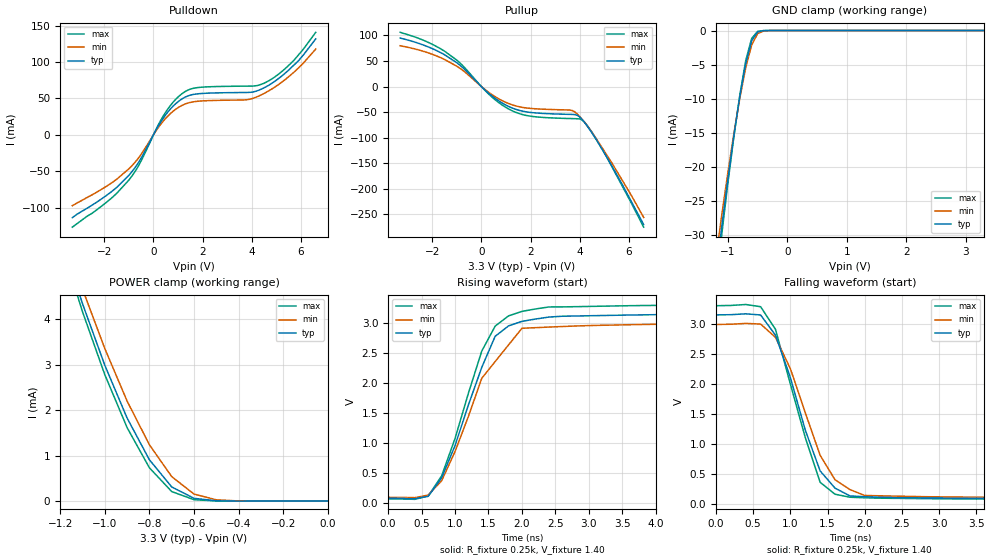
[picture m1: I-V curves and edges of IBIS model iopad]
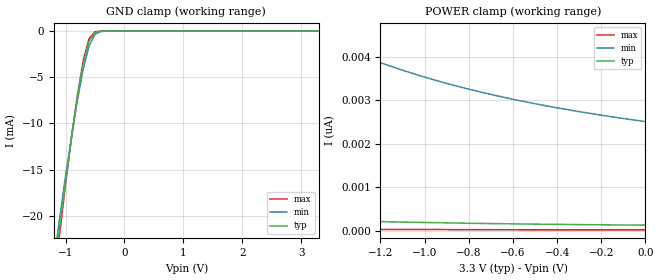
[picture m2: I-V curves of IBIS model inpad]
| IBIS file 70v3579.ibs created by s2ibis2 version 1.1
| North Carolina State University Electronics Research Laboratory  1995
[IBIS ver]   2.1
[File name]   70v3579.ibs
[File Rev]   1.0
[Date]   12/16/98 mff
[Source]   Integrated Device Technology, Inc.
[Notes]   1.Temperatures: typ=25C, min=70C, max=0C 2.RRmp rates based on
   50 ohm load.
[Disclaimer] Integrated Device Technology, Inc. ("IDT") hereby grants the
   user of this IBIS model a non-exclusive, nontransferable
   license to use this IBIS model under the following terms. The
   user is granted this license only to use the IBIS model and is
   not granted rights to sell, copy (except as needed to run the
   IBIS model), rent, lease or sub-license the IBIS model in
   whole or in part, or in modified form to anyone. The User may
   modify the IBIS model to suit its specific applications, but
   rights to derivative works and such modifications shall belong
   to IDT. This IBIS model is provided on an AS IS" basis and IDT
   makes absolutely no warranty with respect to the information
   contained herein. IDT DISCLAIMS AND CUSTOMER WAIVES ALL
   WARRANTIES, EXPRESS AND IMPLIED, INCLUDING WARRANTIES OF
   MERCHANTABILITY AND FITNESS FOR A PARTICULAR PURPOSE. THE
   ENTIRE RISK AS TO QUALITY AND PERFORMANCE IS WITH THE USER
   ACCORDINGLY, IN NO EVENT SHALL IDT BE LIABLE FOR ANY DIRECT OR
   INDIRECT DAMAGES, WHETHER IN CONTRACT OR TORT, INCLUDING ANY
   LOST PROFITS OR OTHER INCIDENTAL, CONSEQUENTIAL, EXEMPLARY, OR
   PUNITIVE DAMAGES ARISING OUT OF THE USE OR APPLICATION OF THE
   IBIS model. Further, IDT reserves the right to make changes
   without notice to any product herein to improve reliability,
   function, or design. IDT does not convey any license under
   patent rights or any other intellectual property rights,
   including those of third parties. IDT is not obligated to
   provide maintenance or support for the licensed IBIS model.
[Copyright]   Copyright 1998, Integrated Device Technology, Inc. all rights
   reserved
|   Component 70v3579dr208
[Component]   70v3579dr208
[Manufacturer]   Integrated Device Technology
[Package]
| variable   typ   min   max
R_pkg   100.00m   50.00m   0.30
L_pkg   12.00nH   10.00nH   14.00nH
C_pkg   2.80pF   1.50pF   6.00pF
[Pin]  signal_name   model_name   R_pin   L_pin   C_pin
1   io19l   iopad
2   io19r   iopad
3   io20l   iopad
4   io20r   iopad
5   vddql   POWER
6   vss   GND
7   io21l   iopad
8   io21r   iopad
9   io22l   iopad
10   io22r   iopad
11   vddqr   POWER
12   vss   GND
13   io23l   iopad
14   io23r   iopad
15   io24l   iopad
16   io24r   iopad
17   vddql   POWER
18   vss   GND
19   io25l   iopad
20   io25r   iopad
21   io26l   iopad
22   io26r   iopad
23   vddqr   POWER
24   vss   GND
25   vdd   POWER
26   vdd   POWER
27   vss   GND
28   vss   GND
29   vddql   POWER
30   vss   GND
31   io27r   iopad
32   io27l   iopad
33   io28r   iopad
34   io28l   iopad
35   vddqr   POWER
36   vss   GND
37   io29r   iopad
38   io29l   iopad
39   io30r   iopad
40   io30l   iopad
41   vddql   POWER
42   vss   GND
43   io31r   iopad
44   io31l   iopad
45   io32r   iopad
46   io32l   iopad
47   vddqr   POWER
48   vss   GND
49   io33r   iopad
50   io33l   iopad
51   io34r   iopad
52   io34l   iopad
53   vss   GND
54   vddql   POWER
55   io35r   iopad
56   io35l   iopad
57   vdd   POWER
58   vss   GND
66   a14r   inpad
67   a13r   inpad
68   a12r   inpad
69   a11r   inpad
70   a10r   inpad
71   a9r   inpad
72   a8r   inpad
73   a7r   inpad
74   be3r#   inpad
75   be2r#   inpad
76   be1r#   inpad
77   be0r#   inpad
78   ce1r   inpad
79   ce0r   inpad
80   vdd   POWER
81   vdd   POWER
82   vss   GND
83   vss   GND
84   clkr   inpad
85   oer#   inpad
86   rwr#   inpad
87   adsr#   inpad
88   cntenr#   inpad
89   cntrstr#   inpad
90   a6r   inpad
91   a5r   inpad
92   a4r   inpad
93   a3r   inpad
94   a2r   inpad
95   a1r   inpad
96   a0r   inpad
97   vdd   POWER
98   vss   GND
99   vss   GND
100   vdd   POWER
101   io0l   iopad
102   io0r   iopad
103   vddql   POWER
104   vss   GND
105   io1l   iopad
106   io1r   iopad
107   io2l   iopad
108   io2r   iopad
109   vddqr   POWER
110   vss   GND
111   io3l   iopad
112   io3r   iopad
113   io4l   iopad
114   io4r   iopad
115   vddql   POWER
116   vss   GND
117   io5l   iopad
118   io5r   iopad
119   io6l   iopad
120   io6r   iopad
121   vddqr   POWER
122   vss   GND
123   io7l   iopad
124   io7r   iopad
125   io8l   iopad
126   io8r   iopad
127   vddql   POWER
128   vss   GND
129   vss   GND
130   vss   GND
131   vdd   POWER
132   vdd   POWER
133   vddqr   POWER
134   vss   GND
135   io9r   iopad
136   io9l   iopad
137   io10r   iopad
138   io10l   iopad
139   vddql   POWER
140   vss   GND
141   io11r   iopad
142   io11l   iopad
143   io12r   iopad
144   io12l   iopad
145   vddqr   POWER
146   vss   GND
147   io13r   iopad
148   io13l   iopad
149   io14r   iopad
150   io14l   iopad
151   vddql   POWER
152   vss   GND
153   io15r   iopad
154   io15l   iopad
155   io16r   iopad
156   io16l   iopad
157   vss   GND
158   vddqr   POWER
159   io17r   iopad
160   io17l   iopad
161   vdd   POWER
162   vss   GND
163   vdd   POWER
164   vdd   POWER
165   a0l   inpad
166   a1l   inpad
167   a2l   inpad
168   a3l   inpad
169   a4l   inpad
170   a5l   inpad
171   a6l   inpad
172   cntrstl#   inpad
173   cntenl#   inpad
174   adsl#   inpad
175   rwl#   inpad
176   oel#   inpad
177   clkl   inpad
178   vss   GND
179   vss   GND
180   vdd   POWER
181   vdd   POWER
182   ce0l   inpad
183   ce1l   inpad
184   be0l#   inpad
185   be1l#   inpad
186   be2l#   inpad
187   be3l#   inpad
188   a7l   inpad
189   a8l   inpad
190   a9l   inpad
191   a10l   inpad
192   a11l   inpad
193   a12l   inpad
194   a13l   inpad
195   a14l   inpad
202   vss   GND
203   vdd   POWER
204   vss   GND
205   io18l   iopad
206   io18r   iopad
207   vddqr   POWER
208   vss   GND
| in   in   dummy_model
| oe   oe   dummy_model
[Pin Mapping]  pulldown_ref   pullup_ref   gnd_clamp_ref   power_clamp_ref
1   vss   vddql
2   vss   vddqr
3   vss   vddql
4   vss   vddqr
5   NC   vddql
6   vss   NC
7   vss   vddql
8   vss   vddqr
9   vss   vddql
10   vss   vddqr
11   NC   vddqr
12   vss   NC
13   vss   vddql
14   vss   vddqr
15   vss   vddql
16   vss   vddqr
17   NC   vddql
18   vss   NC
19   vss   vddql
20   vss   vddqr
21   vss   vddql
22   vss   vddqr
23   NC   vddqr
24   vss   NC
25   NC   vdd
26   NC   vdd
27   vss   NC
28   vss   NC
29   NC   vddql
30   vss   NC
31   vss   vddqr
32   vss   vddql
33   vss   vddqr
34   vss   vddql
35   NC   vddqr
36   vss   NC
37   vss   vddqr
38   vss   vddql
39   vss   vddqr
40   vss   vddql
41   NC   vddql
42   vss   NC
43   vss   vddqr
44   vss   vddql
45   vss   vddqr
46   vss   vddql
47   NC   vddqr
48   vss   NC
49   vss   vddqr
50   vss   vddql
51   vss   vddqr
52   vss   vddql
53   vss   NC
54   NC   vddql
55   vss   vddqr
56   vss   vddql
57   NC   vdd
58   vss   NC
66   vss   vdd
67   vss   vdd
68   vss   vdd
69   vss   vdd
70   vss   vdd
71   vss   vdd
72   vss   vdd
73   vss   vdd
74   vss   vdd
75   vss   vdd
76   vss   vdd
77   vss   vdd
78   vss   vdd
79   vss   vdd
80   NC   vdd
81   NC   vdd
82   vss   NC
83   vss   NC
84   vss   vdd
85   vss   vdd
86   vss   vdd
87   vss   vdd
88   vss   vdd
89   vss   vdd
90   vss   vdd
91   vss   vdd
92   vss   vdd
93   vss   vdd
94   vss   vdd
95   vss   vdd
96   vss   vdd
97   NC   vdd
98   vss   NC
99   vss   NC
100   NC   vdd
101   vss   vddql
102   vss   vddqr
103   NC   vddql
104   vss   NC
105   vss   vddql
106   vss   vddqr
107   vss   vddql
108   vss   vddqr
109   NC   vddqr
110   vss   NC
111   vss   vddql
112   vss   vddqr
113   vss   vddql
114   vss   vddqr
115   NC   vddql
116   vss   NC
117   vss   vddql
118   vss   vddqr
119   vss   vddql
120   vss   vddqr
121   NC   vddqr
122   vss   NC
123   vss   vddql
124   vss   vddqr
125   vss   vddql
126   vss   vddqr
127   NC   vddql
128   vss   NC
129   vss   NC
130   vss   NC
131   NC   vdd
132   NC   vdd
133   NC   vddqr
134   vss   NC
135   vss   vddqr
136   vss   vddql
137   vss   vddqr
138   vss   vddql
139   NC   vddql
140   vss   NC
141   vss   vddqr
142   vss   vddql
143   vss   vddqr
144   vss   vddql
145   NC   vddqr
146   vss   NC
147   vss   vddqr
148   vss   vddql
149   vss   vddqr
150   vss   vddql
151   NC   vddql
152   vss   NC
153   vss   vddqr
154   vss   vddql
155   vss   vddqr
156   vss   vddql
157   vss   NC
158   NC   vddqr
159   vss   vddqr
160   vss   vddql
161   NC   vdd
162   vss   NC
163   NC   vdd
164   NC   vdd
165   vss   vdd
166   vss   vdd
167   vss   vdd
168   vss   vdd
169   vss   vdd
170   vss   vdd
171   vss   vdd
172   vss   vdd
173   vss   vdd
174   vss   vdd
175   vss   vdd
176   vss   vdd
177   vss   vdd
178   vss   NC
179   vss   NC
180   NC   vdd
181   NC   vdd
182   vss   vdd
183   vss   vdd
184   vss   vdd
185   vss   vdd
186   vss   vdd
187   vss   vdd
188   vss   vdd
189   vss   vdd
190   vss   vdd
191   vss   vdd
192   vss   vdd
193   vss   vdd
194   vss   vdd
195   vss   vdd
202   vss   NC
203   NC   vdd
204   vss   NC
205   vss   vddql
206   vss   vddqr
207   NC   vddqr
208   vss   NC
| Models and submodels in the file (2): iopad (I/O), inpad (Input)
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|in   NC   NC
|oe   NC   NC
|   Model iopad
[Model]   iopad
Model_type   I/O
Polarity   Non-Inverting
Enable   Active-High
Vinl =  0.800V
Vinh =  2.000V
Vmeas =  1.500V
C_comp   1.00pF   NA   NA
[Temperature Range]   25.00   70.00   0.000
[Voltage Range]   3.30V   3.15V   3.45V
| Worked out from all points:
|   slope of the pulldown table from 0 to 0.495 V, typ, clamps not added: 18 ohm
|   slope of the pullup table from 0 to 0.495 V, typ, clamps not added: 23.7 ohm
|   GND clamp passes 1 mA (typ) near -0.56 V on its own axis
|   POWER clamp passes 1 mA (typ) near -0.81 V on its own axis
|   rising waveform, R_fixture 0.25k, V_fixture 1.40: 20-80 % time 605ps typ, 716ps min, 576ps max; typ from 0.082 V to 3.15 V
|   falling waveform, R_fixture 0.25k, V_fixture 1.40: 20-80 % time 479ps typ, 525ps min, 448ps max; typ from 3.15 V to 0.082 V
[Pulldown]
| voltage   I(typ)   I(min)   I(max)
-3.3V     -114mA     -97.5mA    -127mA
-1.9V     -83.06mA   -70.53mA   -92.53mA
-1V       -55.69mA   -46.78mA   -62.24mA
-600mV    -37.64mA   -31.5mA    -42.12mA
400mV     22.98mA    18.97mA    26.02mA
1.1V      48.05mA    39.4mA     54.97mA
1.8V      56.39mA    46.16mA    65mA
3.8V      58.27mA    48.27mA    67mA
4.5V      64.64mA    56.89mA    71.01mA
5.1V      77.7mA     69.5mA     83.74mA
5.7V      95.54mA    85.76mA    102mA
6.6V      132mA      118mA      141mA
[Pullup]
| voltage   I(typ)   I(min)   I(max)
-3.3V     94.72mA    79.74mA    106mA
-2.3V     80.13mA    68mA       89.32mA
-1.5V     62.22mA    52.99mA    69.19mA
-800mV    38.7mA     33.19mA    42.88mA
400mV     -17.28mA   -14.82mA   -19.29mA
1.2V      -40.94mA   -34.88mA   -46.19mA
2V        -50.67mA   -42.77mA   -58.01mA
3.6V      -54.45mA   -46.05mA   -62.6mA
4V        -59.66mA   -58.71mA   -63.48mA
4.3V      -76.87mA   -76.45mA   -75.79mA
4.9V      -122mA     -119mA     -121mA
6.6V      -270mA     -256mA     -275mA
[GND_clamp]
| voltage   I(typ)   I(min)   I(max)
-3.3V     -213mA     -195mA     -224mA
-1.2V     -35.67mA   -33.21mA   -37.24mA
-1.1V     -28.54mA   -26.85mA   -29.61mA
-1V       -21.76mA   -20.81mA   -22.35mA
-900mV    -15.43mA   -15.14mA   -15.59mA
-800mV    -9.676mA   -9.946mA   -9.478mA
-700mV    -4.805mA   -5.441mA   -4.393mA
-600mV    -1.485mA   -2.103mA   -1.146mA
-500mV    -215uA     -458uA     -124uA
-400mV    -17.97uA   -58.09uA   -7.861uA
-300mV    -1.106uA   -5.62uA    -349nA
3.3V      143pA      13.86nA    17.08pA
[POWER_clamp]
| voltage   I(typ)   I(min)   I(max)
-3.3V     54.48mA    50.56mA    57.22mA
-1.2V     5.852mA    6.099mA    5.729mA
-1.1V     4.338mA    4.66mA     4.161mA
-1V       2.985mA    3.352mA    2.778mA
-900mV    1.825mA    2.198mA    1.615mA
-800mV    908uA      1.238mA    732uA
-700mV    312uA      538uA      210uA
-600mV    61.42uA    155uA      31.29uA
-500mV    7.539uA    28.27uA    3.013uA
-400mV    726nA      3.93uA     220nA
0V        143pA      2.833nA    18.39pA
[Ramp]
| variable   typ   min   max
dV/dt_r   1.24/1.42n   1.10/1.61n   1.37/1.50n
dV/dt_f   1.37/1.27n   1.20/1.54n   1.50/1.16n
R_load = 50.00
[Rising Waveform]
R_fixture = 0.25k
V_fixture = 1.40
| time   V(typ)   V(min)   V(max)
0s        81.93mV    98.35mV    72.87mV
600ps     115mV      136mV      121mV
800ps     421mV      373mV      454mV
1ns       956mV      858mV      1.074V
1.4ns     2.258V     2.076V     2.528V
1.6ns     2.773V     2.353V     2.942V
1.8ns     2.946V     2.63V      3.112V
2ns       3.021V     2.906V     3.187V
2.4ns     3.092V     2.926V     3.26V
19.8ns    3.148V     2.988V     3.301V
[Falling Waveform]
R_fixture = 0.25k
V_fixture = 1.40
| time   V(typ)   V(min)   V(max)
0s        3.148V     2.988V     3.301V
600ps     3.146V     2.995V     3.284V
800ps     2.81V      2.773V     2.907V
1ns       2.103V     2.251V     1.994V
1.2ns     1.229V     1.519V     1.105V
1.4ns     547mV      807mV      358mV
1.6ns     260mV      400mV      158mV
1.8ns     130mV      236mV      108mV
3.8ns     87.38mV    105mV      76.98mV
19.8ns    81.93mV    98.32mV    72.85mV
|   Model inpad
[Model]   inpad
Model_type   Input
Vinl =  0.800V
Vinh =  2.000V
C_comp   1.00pF   NA   NA
[Temperature Range]   25.00   70.00   0.000
[Voltage Range]   3.30V   3.15V   3.45V
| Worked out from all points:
|   GND clamp passes 1 mA (typ) near -0.59 V on its own axis
[GND_clamp]
| voltage   I(typ)   I(min)   I(max)
-3.3V     -151mA     -139mA     -158mA
-1.2V     -26.48mA   -24.89mA   -27.46mA
-1.1V     -21.24mA   -20.19mA   -21.89mA
-1V       -16.24mA   -15.68mA   -16.56mA
-900mV    -11.52mA   -11.43mA   -11.55mA
-800mV    -7.21mA    -7.515mA   -6.992mA
-700mV    -3.543mA   -4.098mA   -3.185mA
-600mV    -1.064mA   -1.569mA   -793uA
-500mV    -149uA     -338uA     -82.26uA
-400mV    -12.54uA   -43.03uA   -5.213uA
-300mV    -780nA     -4.214uA   -234nA
3.3V      126pA      2.619nA    15.18pA
[POWER_clamp]
| voltage   I(typ)   I(min)   I(max)
-3.3V     884pA      14.8nA     129pA
-2.9V     654pA      11.11nA    94.51pA
-2.5V     486pA      8.384nA    69.46pA
-2V       340pA      6.023nA    47.82pA
-1.6V     262pA      4.75nA     36.18pA
-1.5V     247pA      4.498nA    33.87pA
-1.4V     232pA      4.268nA    31.77pA
-1.2V     208pA      3.867nA    28.12pA
-1V       188pA      3.534nA    25.09pA
-800mV    170pA      3.257nA    22.58pA
-400mV    144pA      2.827nA    18.74pA
0V        126pA      2.51nA     16.01pA
